DATA_BLOCK DB 61
VERSION : 0.1


  STRUCT
   Q11 : INT  := 11;
   Q21 : INT  := 21;
   TEMP1 : REAL  := 2.000000e+000;
   Zeit1 : S5TIME  := S5T#11S;
   Q12 : INT  := 12;
   Q22 : INT  := 22;
   TEMP2 : REAL  := 2.200000e+000;
   Zeit2 : S5TIME  := S5T#12S;
   Q13 : INT  := 13;
   Q23 : INT  := 23;
   TEMP3 : REAL  := 2.300000e+000;
   Zeit3 : S5TIME  := S5T#13S;
   Q14 : INT  := 14;
   Q24 : INT  := 24;
   TEMP4 : REAL  := 2.400000e+000;
   Zeit4 : S5TIME  := S5T#14S;
   Q15 : INT  := 15;
   Q25 : INT  := 25;
   TEMP5 : REAL  := 2.500000e+000;
   Zeit5 : S5TIME  := S5T#15S;
   Q16 : INT  := 16;
   Q26 : INT  := 26;
   TEMP6 : REAL  := 2.600000e+000;
   Zeit6 : S5TIME  := S5T#16S;
   Q17 : INT  := 17;
   Q27 : INT  := 27;
   TEMP7 : REAL  := 2.700000e+000;
   Zeit7 : S5TIME  := S5T#17S;
   Q18 : INT  := 18;
   Q28 : INT  := 28;
   TEMP8 : REAL  := 2.800000e+000;
   Zeit8 : S5TIME  := S5T#18S;
   Q19 : INT  := 19;
   Q29 : INT  := 29;
   TEMP9 : REAL  := 2.900000e+000;
   Zeit9 : S5TIME  := S5T#19S;
   Q110 : INT  := 20;
   Q210 : INT  := 30;
   TEMP10 : REAL  := 3.000000e+000;
   Zeit10 : S5TIME  := S5T#20S;
  END_STRUCT ;
BEGIN
   Q11 := 11;
   Q21 := 21;
   TEMP1 := 2.000000e+000;
   Zeit1 := S5T#11S;
   Q12 := 12;
   Q22 := 22;
   TEMP2 := 2.200000e+000;
   Zeit2 := S5T#12S;
   Q13 := 13;
   Q23 := 23;
   TEMP3 := 2.300000e+000;
   Zeit3 := S5T#13S;
   Q14 := 14;
   Q24 := 24;
   TEMP4 := 2.400000e+000;
   Zeit4 := S5T#14S;
   Q15 := 15;
   Q25 := 25;
   TEMP5 := 2.500000e+000;
   Zeit5 := S5T#15S;
   Q16 := 16;
   Q26 := 26;
   TEMP6 := 2.600000e+000;
   Zeit6 := S5T#16S;
   Q17 := 17;
   Q27 := 27;
   TEMP7 := 2.700000e+000;
   Zeit7 := S5T#17S;
   Q18 := 18;
   Q28 := 28;
   TEMP8 := 2.800000e+000;
   Zeit8 := S5T#18S;
   Q19 := 19;
   Q29 := 29;
   TEMP9 := 2.900000e+000;
   Zeit9 := S5T#19S;
   Q110 := 20;
   Q210 := 30;
   TEMP10 := 3.000000e+000;
   Zeit10 := S5T#20S;
END_DATA_BLOCK

